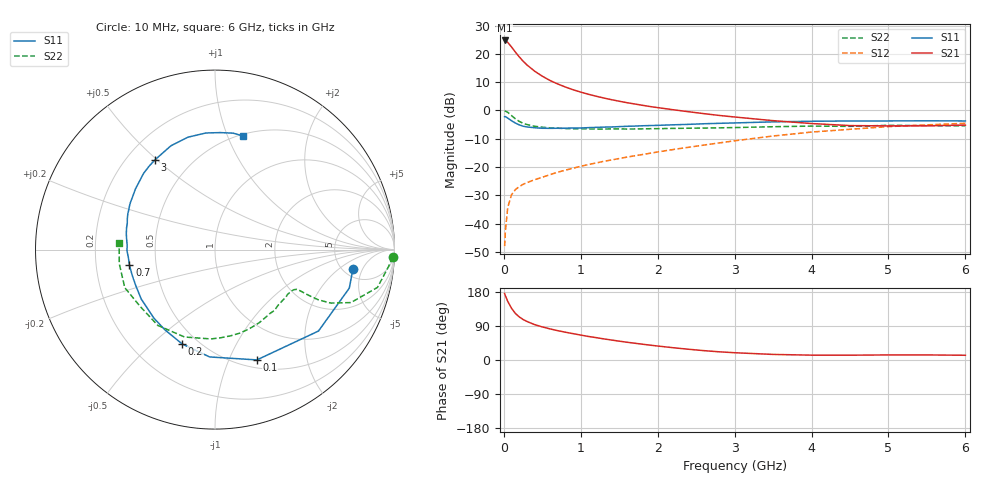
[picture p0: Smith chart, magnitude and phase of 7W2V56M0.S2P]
! Infineon Technologies  Discrete & RF Semiconductors
! BFS17W
! Si NPN RF Bipolar Junction Transistor in SOT323
! VCE = 2.5 V  IC = 6 mA
! Common Emitter S-Parameters:  August  1999
# GHz  S  MA  R  50
!  f  S11  S21  S12  S22
! GHz  MAG  ANG  MAG  ANG  MAG  ANG  MAG  ANG
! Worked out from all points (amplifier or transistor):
!   36 points, 10 MHz to 6 GHz, reference 50 ohm
!   highest |S21| = 24.7 dB at 10 MHz (marker M1)
!   |S21| within 3 dB of that: start of sweep to 119.3 MHz
!   unconditionally stable (mu >= 1): 491.3 MHz to 2.957 GHz; 4.124 GHz to end of sweep
!   at 250 MHz: K = 0.65, MSG = 21.8 dB, |S12| = -26.1 dB
!   at 1.4 GHz: K = 1.26, MAG = 7.6 dB, |S12| = -17.5 dB
!   at 6 GHz: K = 1.09, MAG = -2.1 dB, |S12| = -4.5 dB
!   S11 on the Smith chart (normalised r, x): 10 MHz: 6.13, -3.29; 100 MHz: 0.59, -1.27; 200 MHz: 0.41, -0.63; 700 MHz: 0.35, -0.08; 3 GHz: 0.31, +0.49; 6 GHz: 0.52, +1.14
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0.01  0.776 -7.9  17.24 175.3  0.004 83.7  0.9914 -2.4
0.02  0.7785 -16.0  17.11 169.7  0.0073 84.3  0.9714 -5.6
0.05  0.7337 -38.2  15.97 155.1  0.0191 72.6  0.9294 -13.1
0.1  0.6574 -69.2  13.22 136.4  0.0325 59.8  0.8129 -21.3
0.15  0.5988 -92.9  10.75 122.9  0.0399 52.3  0.71 -24.8
0.2  0.5565 -109.2  8.852 113.8  0.0452 50.2  0.6414 -25.9
0.25  0.5267 -122.1  7.431 107.0  0.0495 48.2  0.594 -26.0
0.3  0.5114 -131.8  6.375 101.7  0.053 48.9  0.5637 -26.0
0.4  0.4947 -146.2  4.943 93.4  0.0597 49.8  0.5248 -25.8
0.5  0.4847 -156.0  4.026 87.3  0.0661 52.2  0.5057 -26.0
0.6  0.483 -163.4  3.385 82.1  0.0733 54.1  0.4934 -26.9
0.7  0.4844 -169.6  2.937 77.5  0.0811 55.8  0.4852 -28.3
0.9  0.4904 -179.2  2.321 69.5  0.0953 58.5  0.475 -31.9
1.1  0.4968 172.7  1.931 62.1  0.1107 60.1  0.4718 -36.3
1.3  0.5077 166.0  1.658 55.7  0.1265 61.6  0.4687 -41.4
1.6  0.5252 157.6  1.371 46.9  0.1497 62.9  0.4694 -49.4
2.2  0.5573 142.7  1.03 32.4  0.2038 64.3  0.4814 -67.3
3  0.6018 123.7  0.766 19.2  0.2909 61.7  0.4983 -92.6
3.5  0.6284 113.0  0.66 14.7  0.3538 57.9  0.5156 -109.2
4.5  0.6517 94.5  0.54 12.7  0.4646 45.8  0.5236 -142.9
5.5  0.6566 81.2  0.535 13.4  0.5564 33.6  0.539 -171.6
6  0.6522 76.0  0.551 12.5  0.5931 27.6  0.5355 175.8
